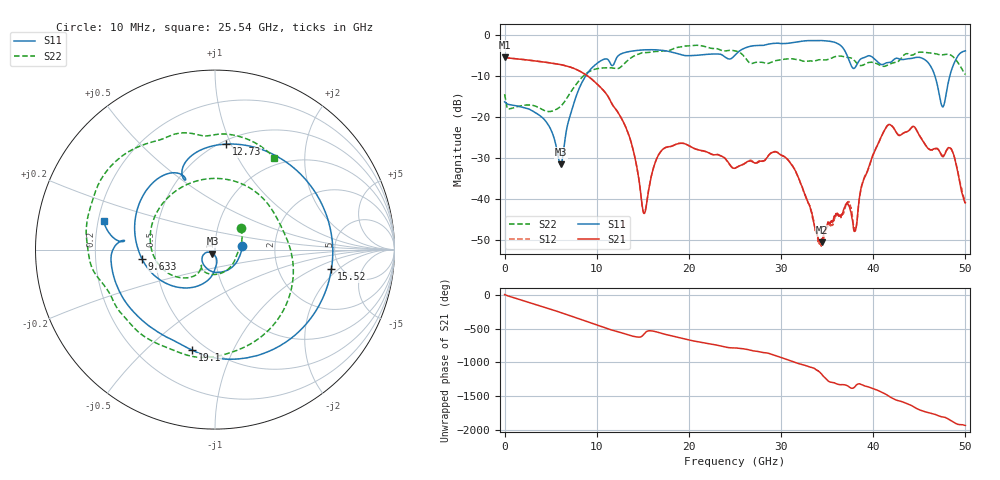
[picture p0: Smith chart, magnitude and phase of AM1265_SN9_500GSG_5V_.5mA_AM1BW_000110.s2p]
!Keysight Technologies,N5245B,MY58422270,A.16.20.02
!Date: Thursday, March 05, 2026 00:30:27
!Correction: S11(C  2-Port  )
!S21(C  2-Port  )
!S12(C  2-Port  )
!S22(C  2-Port  )
!S2P File: Measurements: S11, S21, S12, S22:
# Hz S  dB  R 50
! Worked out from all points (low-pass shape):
!   3201 points, 10 MHz to 50 GHz, reference 50 ohm
!   highest |S21| = -5.51 dB at 10 MHz (marker M1); lowest = -50.7 dB at 34.41 GHz (marker M2)
!   |S21| within 3 dB of the highest: start of sweep to 7.843 GHz
!   lowest |S11| = -31.7 dB at 6.087 GHz (marker M3), VSWR 1.05, Z = 48.6 - j2.13 ohm
!   |S11| at or under -10 dB: start of sweep to 8.818 GHz; 46.69 GHz to 48.31 GHz (1.623 GHz wide, 3.42 % of centre)
!   |S22| runs from -18.8 to -2.5 dB; largest |S21 - S12| = 0.0082
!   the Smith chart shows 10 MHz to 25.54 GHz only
!   S11 on the Smith chart (normalised r, x): 10 MHz: 1.35, +0.05; 9.633 GHz: 0.42, -0.05; 12.73 GHz: 0.53, +0.96; 15.52 GHz: 4.18, -1.63; 19.1 GHz: 0.42, -0.71; 25.54 GHz: 0.22, +0.12
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1e7  -16.36 6.9  -5.51 4.0  -5.54 3.3  -14.49 39.1
2.322038e9  -17.88 -86.1  -6.10 -98.8  -6.10 -98.8  -17.15 -94.1
4.181041e9  -20.37 -138.5  -6.60 -177.9  -6.61 -177.9  -18.33 -129.6
6.086909e9  -31.66 -122.8  -7.26 97.9  -7.27 97.9  -17.48 -126.6
8.352081e9  -11.86 -123.5  -9.10 -8.7  -9.09 -8.6  -10.50 -155.4
9.633075e9  -7.73 -172.8  -11.17 -69.6  -11.15 -69.5  -8.52 161.8
1.124213e10  -6.08 121.2  -15.09 -145.1  -15.08 -145.1  -8.03 85.7
1.272621e10  -4.57 84.1  -20.56 155.3  -20.56 155.3  -7.62 2.3
1.552252e10  -3.64 -9.6  -39.52 -177.3  -39.37 -177.0  -4.33 -114.7
1.667854e10  -3.69 -43.8  -29.44 163.3  -29.45 163.1  -4.05 -141.2
1.909993e10  -4.81 -102.8  -26.49 80.3  -26.49 80.7  -2.95 177.7
2.5005e10  -4.97 173.7  -32.58 -67.2  -32.55 -66.9  -3.91 70.8
2.553614e10  -3.87 165.7  -31.96 -74.0  -31.97 -73.6  -4.33 57.1
3.037892e10  -2.11 82.4  -29.76 133.5  -29.76 133.6  -5.94 -45.7
3.334708e10  -1.39 35.6  -43.55 2.5  -43.43 -5.9  -6.40 -127.7
3.440937e10  -1.39 17.1  -50.69 -95.0  -51.27 -94.0  -6.05 -150.3
3.672141e10  -3.21 -32.1  -43.30 108.4  -43.74 109.0  -5.28 164.5
3.804927e10  -7.95 -25.1  -47.80 84.9  -47.64 -127.6  -6.51 138.5
4.167354e10  -6.78 -54.2  -21.94 -59.7  -21.93 -60.6  -7.30 116.1
4.511035e10  -5.56 -102.3  -24.96 90.7  -24.89 91.2  -4.21 75.8
4.770358e10  -16.88 70.0  -29.44 -13.6  -29.34 -12.9  -4.82 39.9
5e10  -3.91 -73.2  -41.01 -136.2  -40.92 -123.7  -9.71 3.5
